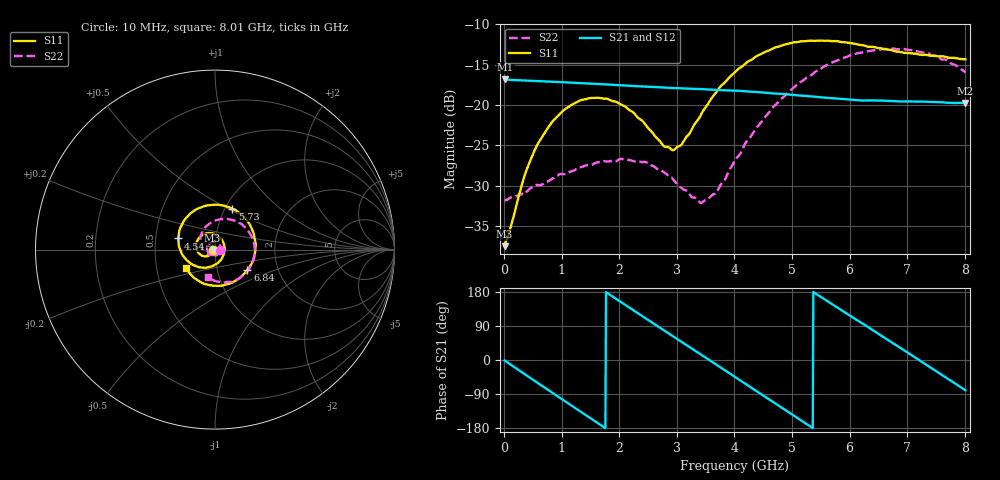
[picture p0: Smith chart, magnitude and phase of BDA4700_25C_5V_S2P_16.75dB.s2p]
!Agilent Technologies,E5071B,MY42404982,A.09.10
!Date: Mon Oct 20 13:34:39 2025
!Data & Calibration Information:
!Freq	S11:SOLT2(ON)	S21:SOLT2(ON)	S12:SOLT2(ON)	S22:SOLT2(ON)
# Hz S RI R 50
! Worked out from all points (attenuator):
!   801 points, 10 MHz to 8.01 GHz, reference 50 ohm
!   highest |S21| = -16.85 dB at 20 MHz (marker M1); lowest = -19.8 dB at 8.01 GHz (marker M2)
!   lowest |S11| = -37.5 dB at 10 MHz (marker M3), VSWR 1.03, Z = 48.7 - j0.154 ohm
!   |S11| at or under -10 dB: start of sweep to end of sweep
!   |S22| runs from -32.1 to -13.0 dB; largest |S21 - S12| = 0.0011
!   S11 on the Smith chart (normalised r, x): 10 MHz: 0.97, -0.00; 4.54 GHz: 0.66, +0.09; 5.73 GHz: 1.08, +0.53; 6.84 GHz: 1.39, -0.33; 8.01 GHz: 0.71, -0.15
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1e7  -0.0133 -0.00158  0.1437 -0.0031  0.1438 -0.00325  0.0257 -0.000884
2e7  -0.0137 -0.0024  0.1437 -0.00553  0.1436 -0.00599  0.0257 -0.00108
3.5e8  -0.0243 -0.0264  0.1139 -0.0841  0.1138 -0.0842  0.0221 -0.0177
5.8e8  -0.0431 -0.0371  0.0701 -0.1217  0.0701 -0.1218  0.0139 -0.0288
8.8e8  -0.075 -0.0327  -0.00173 -0.1389  -0.0017 -0.139  -0.00744 -0.0349
1.35e9  -0.1061 0.0173  -0.1021 -0.0904  -0.1021 -0.0904  -0.0377 -0.017
1.98e9  -0.0518 0.0892  -0.1228 0.0501  -0.1229 0.0501  -0.0329 0.0314
2.45e9  0.0222 0.0726  -0.046 0.1213  -0.046 0.1215  0.000827 0.0444
2.68e9  0.0466 0.0392  0.00485 0.1286  0.00482 0.1286  0.0168 0.036
2.96e9  0.0512 -0.0136  0.0635 0.1101  0.0636 0.11  0.028 0.0191
3.43e9  -0.00743 -0.0882  0.122 0.0286  0.1221 0.0286  0.0177 -0.0173
3.69e9  -0.0663 -0.1005  0.1209 -0.0272  0.1209 -0.0275  -0.00257 -0.0285
4.01e9  -0.1421 -0.0723  0.0871 -0.0863  0.0871 -0.0862  -0.0364 -0.0267
4.54e9  -0.2044 0.062  -0.0165 -0.118  -0.0164 -0.1181  -0.0799 0.0284
4.9e9  -0.1663 0.1696  -0.0807 -0.0839  -0.0806 -0.0842  -0.0752 0.0887
5.35e9  -0.0379 0.2468  -0.1128 -0.00264  -0.1128 -0.00297  -0.0131 0.1536
5.73e9  0.0959 0.2289  -0.0889 0.0646  -0.0888 0.0647  0.0734 0.1699
6.22e9  0.2116 0.1006  -0.0121 0.1057  -0.0111 0.1061  0.1814 0.1084
6.68e9  0.2104 -0.0636  0.0661 0.0827  0.0663 0.0828  0.2212 -0.00839
6.84e9  0.1805 -0.1142  0.0854 0.0616  0.0857 0.0611  0.2145 -0.0531
7.41e9  0.0063 -0.2017  0.0979 -0.0364  0.098 -0.0367  0.1161 -0.1672
8.01e9  -0.1606 -0.1049  0.0178 -0.1011  0.0181 -0.1012  -0.0367 -0.1546
